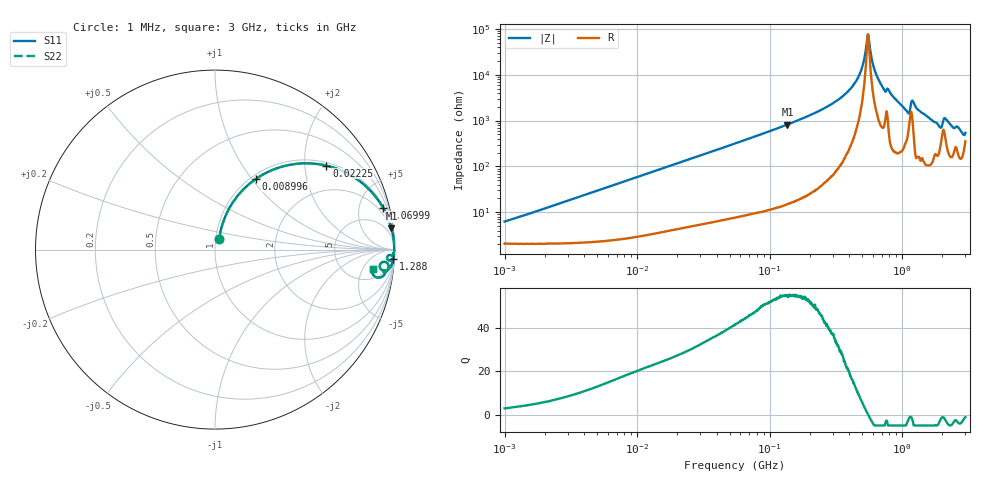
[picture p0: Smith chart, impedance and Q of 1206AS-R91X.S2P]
!s-Parameter Generated by FASTRON Sdn. Bhd.
!FASTRON P/N : 1206AS-R91X
!Keysight Technologies: E4991B_MY54100416_A.01.15
!Date created: Thu Nov 16 13:33:52 2023
!Version  : Rev00 Thu Nov 16 13:33:52 2023
!Data & Calibration Information:
!Freq	S11	S21	S12	S22
!PortZ  Port1:50+j0  Port2:50+j0
!When reading reference impedance value at option line is always used.
! Remarks : This data is being provided solely for informational purposes.
# Hz S dB R 50
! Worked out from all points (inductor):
!   1601 points, 1 MHz to 3 GHz, reference 50 ohm
!   read as one part in series: L = 942 nH near 1.057 MHz
!   highest Q = 54.8 at 136.2 MHz (marker M1), where L = 958 nH
!   self-resonance near 550.1 MHz
!   S11 on the Smith chart (normalised r, x): 1 MHz: 1.04, +0.12; 8.996 MHz: 1.06, +1.06; 22.25 MHz: 1.09, +2.58; 69.99 MHz: 1.18, +8.10; 1.288 GHz: 4, -37; 3 GHz: 8, -8
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1000000  -24.24 67.4  -0.19 -3.3  -0.19 -3.3  -24.24 67.4
3804036  -13.33 72.1  -0.39 -12.4  -0.39 -12.4  -13.33 72.1
8995704  -6.80 59.8  -1.25 -27.2  -1.25 -27.2  -6.80 59.8
1.447069e7  -3.98 48.4  -2.51 -39.2  -2.51 -39.2  -3.98 48.4
2.225279e7  -2.19 37.0  -4.40 -51.0  -4.40 -51.0  -2.19 37.0
5.477226e7  -0.47 17.4  -10.47 -71.2  -10.47 -71.2  -0.47 17.4
6.999185e7  -0.30 13.8  -12.45 -75.0  -12.45 -75.0  -0.30 13.8
1.361705e8  -0.08 6.9  -18.36 -82.0  -18.36 -82.0  -0.08 6.9
2.083556e8  -0.04 4.2  -22.75 -84.7  -22.75 -84.7  -0.04 4.2
3.204059e8  -0.02 2.1  -28.63 -86.1  -28.63 -86.1  -0.02 2.1
4.198105e8  -0.01 1.0  -34.80 -85.4  -34.80 -85.4  -0.01 1.0
4.878085e8  -0.01 0.5  -41.59 -81.2  -41.59 -81.2  -0.01 0.5
5.500551e8  -0.01 0.0  -57.45 -12.9  -57.45 -12.9  -0.01 0.0
6.488164e8  -0.01 -0.6  -39.04 81.0  -39.04 81.0  -0.01 -0.6
7.243229e8  -0.03 -1.1  -33.86 80.6  -33.86 80.6  -0.03 -1.1
7.925923e8  -0.02 -1.2  -33.18 81.9  -33.18 81.9  -0.02 -1.2
1.086329e9  -0.15 -3.4  -24.17 72.6  -24.17 72.6  -0.15 -3.4
1.200675e9  -0.11 -2.0  -28.70 68.5  -28.70 68.5  -0.11 -2.0
1.287806e9  -0.05 -3.1  -25.37 82.1  -25.37 82.1  -0.05 -3.1
1.902655e9  -0.37 -7.0  -17.90 67.4  -17.90 67.4  -0.37 -7.0
2.124078e9  -0.30 -4.7  -21.17 64.9  -21.17 64.9  -0.30 -4.7
3e9  -1.06 -7.1  -15.68 42.0  -15.68 42.0  -1.06 -7.1
